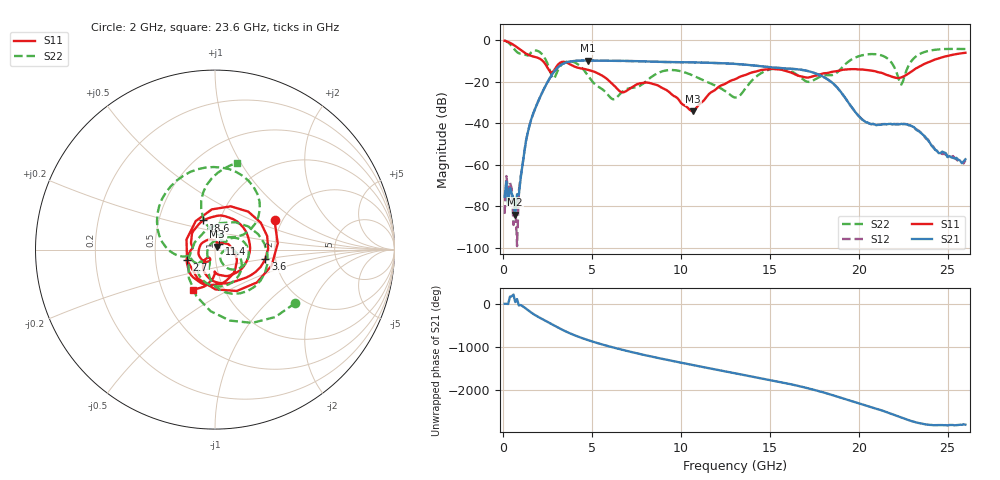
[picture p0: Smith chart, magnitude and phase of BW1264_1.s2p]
!Keysight Technologies,N5245B,MY57181159,A.13.60.06
!Date: Friday, December 18, 2020 23:51:57
!Correction: S11(Full 2 Port(1,2))
!S21(Full 2 Port(1,2))
!S12(Full 2 Port(1,2))
!S22(Full 2 Port(1,2))
!S2P File: Measurements: S11, S21, S12, S22:
# Hz S  dB  R 50
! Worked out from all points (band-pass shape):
!   260 points, 100 MHz to 26 GHz, reference 50 ohm
!   highest |S21| = -9.84 dB at 4.8 GHz (marker M1); lowest = -83.9 dB at 700 MHz (marker M2)
!   |S21| within 3 dB of the highest: 3.136 GHz to 14.77 GHz (11.63 GHz wide, 130 % of centre)
!   lowest |S11| = -34.3 dB at 10.7 GHz (marker M3), VSWR 1.04, Z = 51.1 + j1.61 ohm
!   |S11| at or under -10 dB: 2.236 GHz to 24.1 GHz (21.87 GHz wide, 166 % of centre)
!   |S22| runs from -28.5 to -0.2 dB; largest |S21 - S12| = 0.0006
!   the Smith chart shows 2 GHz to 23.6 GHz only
!   S11 on the Smith chart (normalised r, x): 2 GHz: 1.83, +0.69; 2.7 GHz: 0.73, -0.09; 3.6 GHz: 1.76, -0.21; 11.4 GHz: 1.05, +0.07; 18.6 GHz: 0.84, +0.28; 23.6 GHz: 0.71, -0.34
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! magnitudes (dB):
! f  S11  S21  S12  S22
! 100 MHz  -0.3  -75.5  -83.6  -0.2
! 200 MHz  -0.6  -68.0  -65.4  -0.6
! 300 MHz  -0.9  -79.4  -72.7  -1.2
! 400 MHz  -1.3  -71.0  -68.5  -1.9
! 700 MHz  -2.9  -83.9  -78.5  -4.9
! 2 GHz  -8.7  -29.2  -29.3  -5.4
! 2.7 GHz  -15.6  -17.5  -17.5  -16.0
! 3.6 GHz  -10.9  -10.7  -10.7  -10.4
! 4.5 GHz  -13.8  -9.9  -9.9  -13.9
! 4.8 GHz  -14.4  -9.8  -9.8  -17.3
! 6.2 GHz  -21.4  -10.0  -10.0  -28.5
! 8.8 GHz  -22.2  -10.5  -10.5  -15.5
! 10.7 GHz  -34.3  -10.7  -10.7  -17.1
! 11.4 GHz  -27.9  -10.9  -10.9  -19.8
! 13.1 GHz  -18.7  -11.5  -11.5  -27.6
! 15.1 GHz  -13.9  -13.1  -13.1  -14.0
! 17.4 GHz  -17.5  -15.5  -15.5  -19.7
! 18.6 GHz  -15.1  -21.2  -21.1  -16.7
! 21.7 GHz  -17.1  -40.3  -40.5  -9.4
! 22.4 GHz  -18.0  -40.3  -40.5  -21.4
! 23.6 GHz  -11.9  -45.4  -45.4  -6.0
! 26 GHz  -6.1  -57.3  -57.8  -4.3
